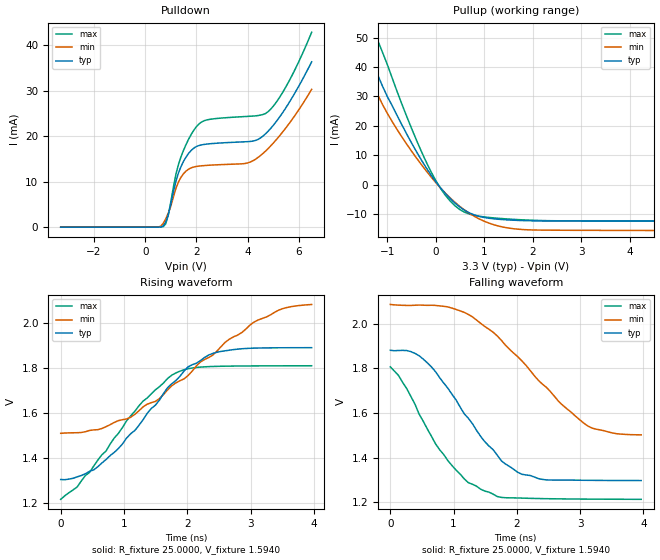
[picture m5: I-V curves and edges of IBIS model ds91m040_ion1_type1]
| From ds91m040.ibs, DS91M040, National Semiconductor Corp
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|   Model ds91m040_ion1_type1
[Model]  ds91m040_ion1_type1
Model_type I/O
Polarity   Inverting
Vinl = -0.05
Vinh = 0.05
Vmeas =  1.56V
Rref =   25.0000
Vref =   1.56V
C_comp   7.359p   6.991p  7.743p
[Model Spec]
S_overshoot_high   3.8   3.8   3.8
S_overshoot_low   -1.4   -1.4   -1.4
[Temperature Range]   25.0000   85.0000   -40.0000
[Voltage Range]   3.3000V   3.0000V   3.6000V
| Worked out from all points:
|   slope of the pullup table from 0 to 0.495 V, typ, clamps not added: 57.8 ohm
|   rising waveform, R_fixture 25.0000, V_fixture 1.5940: 20-80 % time 1.08ns typ, 1.61ns min, 1ns max; typ from 1.3 V to 1.89 V
|   falling waveform, R_fixture 25.0000, V_fixture 1.5940: 20-80 % time 916ps typ, 1.2ns min, 785ps max; typ from 1.88 V to 1.3 V
[Pulldown]
|Voltage   I(typ)   I(min)   I(max)
-3.3V     -16.04uA   -15.04uA   -17.07uA
500mV     -2.06uA    10.82uA    -4.562uA
700mV     234.6uA    784.7uA    91.14uA
900mV     2.713mA    3.039mA    2.586mA
1.2V      10.09mA    8.499mA    11.63mA
1.4V      13.34mA    10.98mA    15.49mA
2V        17.72mA    13.33mA    22.08mA
2.5V      18.31mA    13.61mA    23.68mA
4V        18.79mA    14.11mA    24.35mA
4.8V      21.08mA    17.27mA    25.39mA
5.6V      27.19mA    22.62mA    31.92mA
6.5V      36.35mA    30.31mA    42.84mA
[Pullup]
|Voltage   I(typ)   I(min)   I(max)
-3.3V     175.7mA    142.4mA    190.6mA
-1.7V     63.82mA    53.26mA    77.6mA
-1.5V     51.44mA    43.29mA    64.96mA
-1.3V     41.45mA    34.36mA    54.06mA
-800mV    23.56mA    18.75mA    31.69mA
-400mV    11.23mA    9.085mA    15.15mA
-100mV    3.299mA    2.667mA    4.432mA
200mV     -3.058mA   -2.926mA   -3.666mA
600mV     -8.75mA    -8.684mA   -9.419mA
1.2V      -11.61mA   -13.63mA   -11.3mA
1.8V      -12.2mA    -15.25mA   -11.96mA
6.5V      -12.39mA   -15.63mA   -12.32mA
[Ramp]
| variable   typ   min   max
dV/dt_r  0.3567/1.100n   0.3514/1.640n   0.3599/1.010n
dV/dt_f  0.3578/0.936n   0.3457/1.180n   0.3610/0.798n
R_load = 25.00
[Rising Waveform]
R_fixture= 25.0000
V_fixture= 1.5940
V_fixture_min= 1.7950
V_fixture_max= 1.5120
|time   V(typ)   V(min)   V(max)
0s        1.303V     1.509V     1.215V
260ps     1.315V     1.512V     1.27V
585ps     1.36V      1.526V     1.389V
1.3ns     1.569V     1.627V     1.652V
1.82ns    1.745V     1.734V     1.779V
2.015ns   1.806V     1.768V     1.798V
2.47ns    1.871V     1.876V     1.808V
3.12ns    1.89V      2.015V     1.81V
3.51ns    1.891V     2.066V     1.81V
3.965ns   1.891V     2.084V     1.811V
[Falling Waveform]
R_fixture= 25.0000
V_fixture= 1.5940
V_fixture_min= 1.7950
V_fixture_max= 1.5120
|time   V(typ)   V(min)   V(max)
0s        1.881V     2.086V     1.807V
260ps     1.88V      2.082V     1.71V
585ps     1.825V     2.082V     1.529V
975ps     1.684V     2.07V      1.365V
1.43ns    1.495V     2.001V     1.259V
1.755ns   1.386V     1.926V     1.223V
2.08ns    1.326V     1.833V     1.219V
2.665ns   1.3V       1.651V     1.216V
3.12ns    1.299V     1.542V     1.215V
3.965ns   1.298V     1.502V     1.214V
